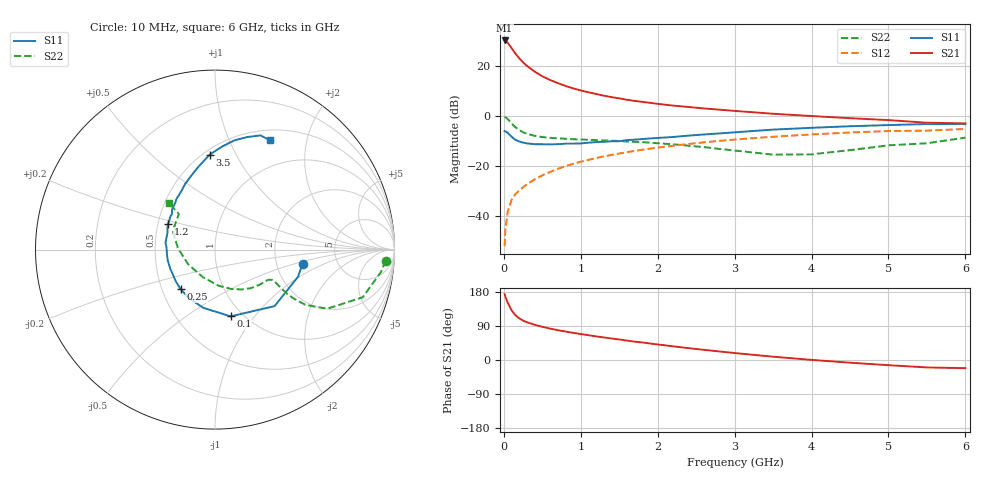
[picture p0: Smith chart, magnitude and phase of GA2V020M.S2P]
! Infineon Technologies  Discrete & RF Semiconductors
! BF775
! Si NPN RF Bipolar Junction Transistor in SOT23
! VCE = 2 V  IC = 20 mA
! Common Emitter S-Parameters:  May  1996
# GHz  S  MA  R  50
!  f  S11  S21  S12  S22
! GHz  MAG  ANG  MAG  ANG  MAG  ANG  MAG  ANG
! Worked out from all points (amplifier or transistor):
!   36 points, 10 MHz to 6 GHz, reference 50 ohm
!   highest |S21| = 30.1 dB at 10 MHz (marker M1)
!   |S21| within 3 dB of that: start of sweep to 99.18 MHz
!   unconditionally stable (mu >= 1): 335.8 MHz to 3.706 GHz; 5.385 GHz to 5.809 GHz
!   at 250 MHz: K = 0.92, MSG = 24.9 dB, |S12| = -28.5 dB
!   at 1.4 GHz: K = 1.14, MAG = 9.2 dB, |S12| = -15.6 dB
!   at 6 GHz: K = 1.00, MSG = 1.1 dB, |S12| = -5.3 dB
!   S11 on the Smith chart (normalised r, x): 10 MHz: 2.81, -0.59; 100 MHz: 0.88, -0.77; 250 MHz: 0.62, -0.30; 1.2 GHz: 0.56, +0.18; 3.5 GHz: 0.54, +0.79; 6 GHz: 0.63, +1.43
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0.01  0.494 -9.3  31.85 173.8  0.0025 92.4  0.9529 -3.7
0.02  0.4869 -18.1  31.3 167.6  0.0054 82.8  0.9329 -7.7
0.05  0.4575 -43.5  28.72 151.2  0.0121 74.4  0.8647 -17.9
0.1  0.382 -76.8  22.46 131.4  0.0209 66.7  0.7065 -27.8
0.15  0.3312 -101.1  17.46 118.3  0.0274 64.3  0.5917 -31.4
0.2  0.3074 -117.9  14.07 110.0  0.0321 65.1  0.5179 -31.9
0.25  0.2919 -131.1  11.64 104.0  0.0375 65.7  0.4684 -31.4
0.3  0.2811 -140.8  9.915 99.6  0.0431 67.1  0.4377 -30.6
0.4  0.271 -156.2  7.627 93.1  0.0537 68.4  0.399 -29.1
0.5  0.2702 -166.6  6.149 87.5  0.0647 69.3  0.3763 -28.1
0.6  0.2689 -174.4  5.196 82.9  0.0756 69.5  0.3634 -27.9
0.7  0.2704 177.5  4.495 78.8  0.0873 69.4  0.3552 -28.3
0.8  0.2783 172.1  3.949 75.2  0.0983 68.9  0.3475 -28.9
0.9  0.2783 166.0  3.53 71.7  0.1099 68.2  0.3409 -29.7
1.1  0.2904 156.1  2.941 65.5  0.1319 66.8  0.3317 -32.5
1.2  0.2985 151.5  2.721 62.3  0.1434 65.8  0.3263 -33.8
1.6  0.3272 137.0  2.087 51.2  0.188 61.5  0.307 -41.1
2.2  0.3775 119.5  1.596 36.1  0.2528 54.3  0.2699 -55.3
3.5  0.5299 93.2  1.098 8.7  0.3817 36.4  0.1677 -113.7
4.5  0.6184 79.9  0.895 -7.1  0.4639 22.5  0.2062 178.2
5.5  0.6848 68.3  0.727 -19.6  0.5049 7.8  0.2828 135.4
6  0.6818 63.4  0.705 -21.6  0.546 3.6  0.3668 134.7
